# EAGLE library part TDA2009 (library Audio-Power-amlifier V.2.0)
Power OP AMP
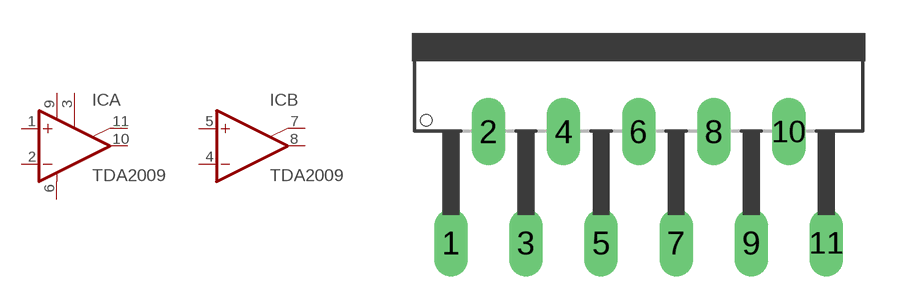
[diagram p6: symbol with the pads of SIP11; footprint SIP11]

Designator prefix IC; gates A=2005 B=2005A

## TDA2009T  [SIP11]
1  A:+IN  in
2  A:-IN  in
3  A:SVRR  pas
4  B:-IN  in
5  B:+IN  in
6  A:GND  pwr
7  B:BTSP  pas
8  B:OUT  out
9  A:V+  pwr
10  A:OUT  out
11  A:BTSP  pas

## Footprint SIP11 (pad centres in mm)
TO-220 11 lead, National Semiconductor
drill 1.016 long: 1 -8.509,-9.525; 2 -6.807,-4.47; 3 -5.105,-9.525; 4 -3.404,-4.47; 5 -1.702,-9.525; 6 0,-4.47; 7 1.702,-9.525; 8 3.404,-4.47; 9 5.105,-9.525; 10 6.807,-4.47; 11 8.509,-9.525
